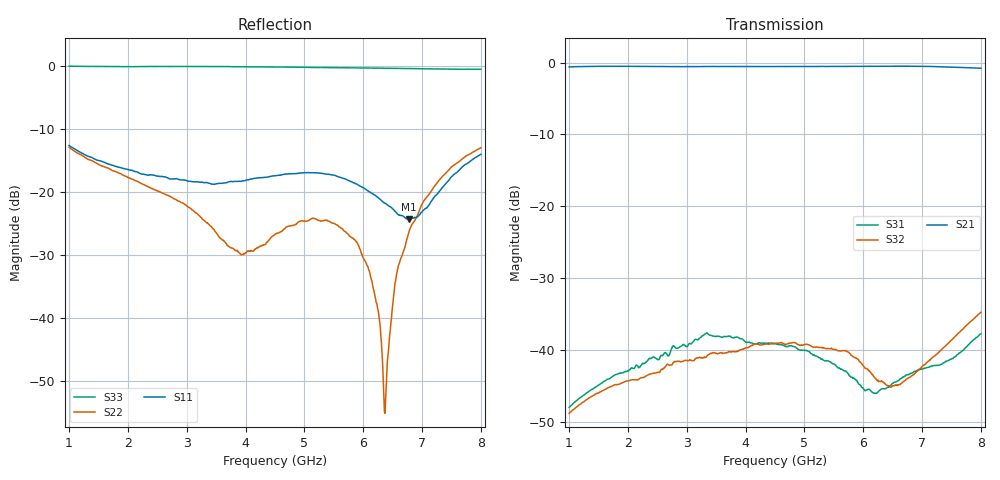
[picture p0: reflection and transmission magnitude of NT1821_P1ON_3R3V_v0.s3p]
! NT1821 PC-P1 ON state
! Port1:PC, Port2:P1, Port3:P2
! VDD=3.3V, VCTL=1.2V
# hz S ma R 50
! 3 Port Network Data from SP1.SP block
! freq  magS11  angS11  magS12  angS12  magS13  angS13
!  magS21  angS21
!  magS22  angS22  magS23  angS23
!  magS31  angS31  magS32  angS32
!  magS33  angS33
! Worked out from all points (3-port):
!   701 points, 1 GHz to 8 GHz, reference 50 ohm
!   strongest paths, dB at 1 GHz, 2.75 GHz, 4.5 GHz, 6.25 GHz, 8 GHz:
!     S21: -0.6, -0.6, -0.6, -0.5, -0.8
!     S32: -48.8, -42.1, -39.1, -44.2, -34.8
!     S31: -48.0, -39.7, -39.1, -45.9, -37.8
!   lowest |S11| = -24.3 dB at 6.77 GHz (marker M1), VSWR 1.13, Z = 48 - j5.66 ohm
!   |S11| at or under -10 dB: start of sweep to end of sweep
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1e9  0.2354 -77.3  0.9336 2.0  0.003977 75.4
     0.9322 1.9  0.2276 -77.7  0.003623 71.8
     0.003978 75.4  0.003616 71.7  1.003 -13.3
3.93e9  0.1225 -40.2  0.9402 -33.6  0.01195 51.0
        0.9382 -33.7  0.03173 -178.0  0.01004 63.9
        0.01192 50.7  0.01002 63.6  0.9933 -42.0
4.5e9  0.135 -32.0  0.939 -39.5  0.01107 49.8
       0.9376 -39.5  0.0462 118.7  0.01106 57.7
       0.01107 49.2  0.0111 57.2  0.9879 -49.6
5.16e9  0.1428 -31.6  0.9395 -46.0  0.009237 44.7
        0.9379 -45.8  0.06213 91.7  0.01045 52.1
        0.009258 44.2  0.01044 51.5  0.9787 -61.6
5.89e9  0.1161 -43.0  0.9413 -53.1  0.006072 52.7
        0.9401 -53.1  0.03998 80.8  0.008715 47.8
        0.006138 51.4  0.008676 47.1  0.9725 -78.6
6.24e9  0.09176 -55.6  0.9428 -56.7  0.005059 78.7
        0.9412 -56.8  0.01222 76.5  0.006086 57.9
        0.005046 77.9  0.006105 57.5  0.9683 -87.2
6.37e9  0.08173 -63.7  0.9435 -58.2  0.005332 85.5
        0.9422 -58.2  0.001751 -177.1  0.005803 66.4
        0.005352 85.2  0.005824 66.0  0.9665 -90.4
6.55e9  0.06965 -78.7  0.9439 -60.2  0.005991 94.8
        0.9426 -60.1  0.01989 -117.0  0.005678 82.3
        0.005961 93.7  0.005705 82.0  0.9646 -94.5
6.77e9  0.06114 -106.1  0.9436 -62.7  0.006779 101.7
        0.9423 -62.6  0.04706 -116.1  0.006367 98.4
        0.00675 101.2  0.006397 97.6  0.9606 -99.2
8e9  0.2003 166.8  0.9139 -76.4  0.013 135.6
     0.9124 -76.4  0.2256 -122.2  0.01823 127.6
     0.01295 135.0  0.01825 127.3  0.9473 -116.5
